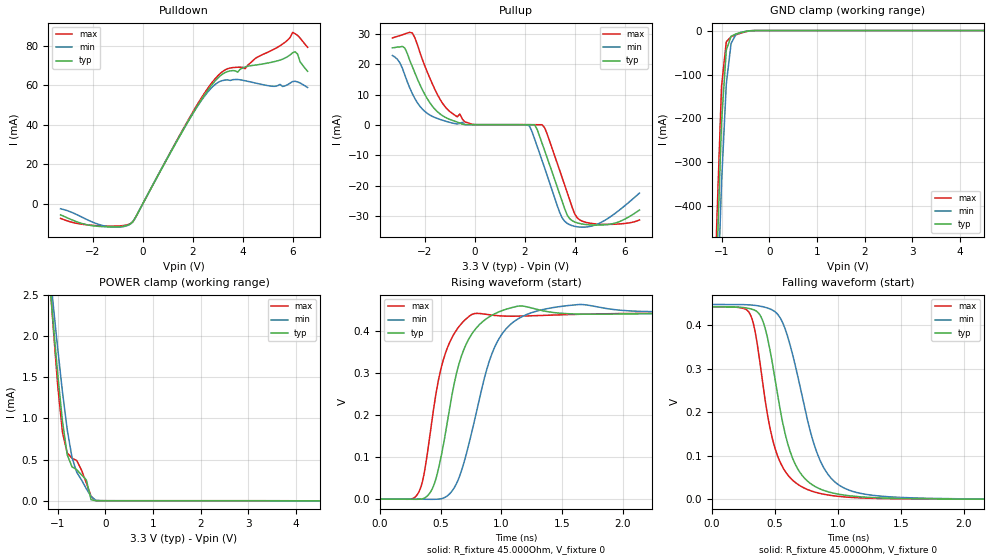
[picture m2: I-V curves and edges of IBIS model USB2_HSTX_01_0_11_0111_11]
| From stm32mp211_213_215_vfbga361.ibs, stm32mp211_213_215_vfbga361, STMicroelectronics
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[Model] USB2_HSTX_01_0_11_0111_11
Model_type   Output
Polarity   Non-Inverting
Enable   Active-High
C_comp   8.036pF   7.631pF   8.569pF
Vmeas = 200.000mV
Vref = 200.000mV
Rref = 45Ohms
Cref = 0pF
[Model Spec]
Vmeas   200.000mV   200.000mV   200.000mV
Vref   200.000mV   200.000mV   200.000mV
| This model is not intended for timing simulations.
| Warnings about Cref, Vref & Rref can be ignored
[Temperature Range]   25.000   125.000   -40.000
[Voltage Range]   3.300V   3.070V   3.630V
[GND Clamp Reference]   0.00V   0.00V   0.00V
[Pulldown Reference]   0.00V   0.00V   0.00V
[POWER Clamp Reference]   3.300V   3.070V   3.630V
[Pullup Reference]   3.300V   3.070V   3.630V
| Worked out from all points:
|   slope of the pulldown table from 0 to 0.495 V, typ, clamps not added: 42.6 ohm
|   GND clamp passes 1 mA (typ) near -0.43 V on its own axis
|   POWER clamp passes 1 mA (typ) near -0.91 V on its own axis
|   rising waveform, R_fixture 45.000Ohm, V_fixture 0: 20-80 % time 194ps typ, 246ps min, 168ps max; typ from 0 V to 0.442 V
|   falling waveform, R_fixture 45.000Ohm, V_fixture 0: 20-80 % time 196ps typ, 242ps min, 176ps max; typ from 0.442 V to 0 V
[GND Clamp]
-3.3V     -11.02A    -10.62A    -11.32A
-1.2V     -931.6mA   -1.049A    -855.7mA
-1.1V     -533.1mA   -671.7mA   -440.2mA
-1V       -209.4mA   -347mA     -127.3mA
-900mV    -44.44mA   -121.7mA   -25.6mA
-800mV    -13.15mA   -29.48mA   -14.15mA
-700mV    -7.743mA   -9.125mA   -9.769mA
-500mV    -2.127mA   -1.981mA   -2.894mA
-300mV    -19.54uA   -62.22uA   -13.65uA
6.6V      10.37uA    26.59uA    21.05uA
[Power Clamp]
-3.3V     3.206A     2.175A     4.855A
-1.2V     2.88mA     3.008mA    2.969mA
-1.1V     2.195mA    2.419mA    2.156mA
-1V       1.545mA    1.852mA    1.406mA
-900mV    967.9uA    1.324mA    831.4uA
-800mV    558.5uA    864.6uA    580.3uA
-700mV    412uA      525.9uA    517uA
-600mV    376.6uA    345uA      488.5uA
-400mV    254.2uA    146.6uA    216.8uA
-300mV    11.21uA    52.87uA    53.51uA
-100mV    94.74nA    985nA      361.1nA
6.6V      -2.4uA     -5.18uA    -3.523uA
[Pulldown]
-3.3V     -5.671mA   -2.581mA   -7.449mA
-1.6V     -11.64mA   -11.09mA   -11.31mA
-500mV    -10.25mA   -10.32mA   -10.1mA
1.9V      43.42mA    43.46mA    44.13mA
2.9V      62.15mA    60.37mA    63.26mA
3.4V      66.87mA    62.63mA    68.29mA
4.1V      69.19mA    62.19mA    68.26mA
4.5V      70.11mA    61.06mA    73.4mA
5.6V      73.12mA    59.29mA    80.76mA
6V        76.33mA    61.79mA    86.69mA
6.1V      76.87mA    61.93mA    85.99mA
6.6V      66.99mA    58.79mA    79.1mA
[Pullup]
-3.3V     25.41mA    22.87mA    28.69mA
-2.8V     25.3mA     16.38mA    30mA
-2.5V     19.22mA    10.28mA    30.28mA
-1.7V     6.185mA    2.829mA    13.54mA
-1.2V     2.602mA    1.31mA     6.111mA
-400mV    111.7uA    77.66uA    1.021mA
2.2V      68.69uA    -465.1uA   104.8uA
2.4V      56.19uA    -4.685mA   90.82uA
2.8V      -8.459mA   -14.22mA   -920uA
3.7V      -29.65mA   -32.41mA   -22.19mA
4.3V      -32.64mA   -33.68mA   -31.68mA
6.6V      -28.04mA   -22.46mA   -31.3mA
[Ramp]
R_load=45.000Ohm
dV/dt_r   633.011mV/985.000ps  601.227mV/995.000ps  686.726mV/930.000ps
dV/dt_f   635.188mV/225.000ps  604.110mV/285.000ps  688.529mV/210.000ps
[Rising waveform]
R_fixture=45.000Ohm
V_fixture=0
0s        452.2nV    3.135uV    468.1nV
330ps     -324.5uV   -446.7uV   23.59mV
460ps     47.91mV    -503.1uV   249.5mV
590ps     243.5mV    18.03mV    382.6mV
670ps     339.7mV    66.35mV    417.2mV
770ps     398.4mV    176.3mV    440.7mV
940ps     440.1mV    358.5mV    437mV
1.14ns    459.1mV    429.2mV    435.1mV
1.65ns    440mV      462.9mV    439.7mV
9.9ns     442.4mV    448.1mV    442.6mV
[Falling waveform]
R_fixture=45.000Ohm
V_fixture=0
0s        441.9mV    447.5mV    442.1mV
310ps     437.2mV    446.4mV    421mV
420ps     395.5mV    441.2mV    232.6mV
530ps     225.9mV    422mV      93.32mV
680ps     70.6mV     285.1mV    34.83mV
810ps     31.07mV    127.6mV    17.26mV
930ps     16.7mV     54.26mV    9.582mV
1.17ns    6.018mV    14.36mV    3.408mV
1.75ns    988.7uV    2.168mV    757.9uV
9.9ns     14.43uV    30.88uV    4.971uV
